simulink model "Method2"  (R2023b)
settings: Solver=FixedStepDiscrete  StartTime=0.0  StopTime=0.5  RelTol=1e-3  EnableMultiTasking=on
undefined symbols (not defined in the file): Datasheet, derived, set
libraries: fl_lib x13, nesl_utility x9, ee_lib x4, slpidlib x1, simulink x1, simulink_extras x1, spspowerguiLib x1

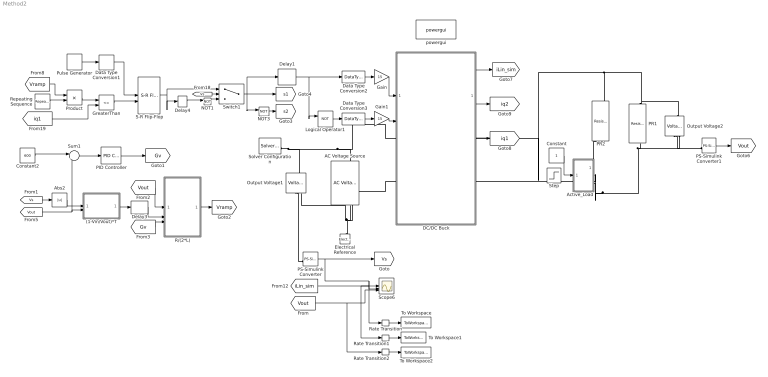
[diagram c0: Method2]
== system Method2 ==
  (1-Vin/Vout)*T : MATLAB Function  TreatAsAtomicUnit=on
  AC Voltage Source : fl_lib/Electrical/Electrical Sources/AC Voltage Source  amp=340 V  shift=0 deg  frequency=50 Hz  omega=0 rad/s
  Abs2 : Abs
  Active_Load : Subsystem
  Constant : Constant
  Constant2 : Constant  Value=600
  DC/DC Buck : Subsystem
  Data Type Conversion1 : DataTypeConversion
  Data Type Conversion2 : DataTypeConversion  OutDataTypeStr=double  RndMeth=Simplest
  Data Type Conversion3 : DataTypeConversion  OutDataTypeStr=double  RndMeth=Simplest
  Delay1 : Delay  DelayLength=1
  Delay3 : Delay  DelayLength=10
  Delay4 : Delay  DelayLength=100e3
  Electrical Reference : fl_lib/Electrical/Electrical Elements/Electrical Reference
  Gain : Gain  Gain=15
  Gain1 : Gain  Gain=15
  GreaterThan : RelationalOperator  Operator=<=  OutDataTypeStr=boolean  RndMeth=Simplest
  Logical Operator1 : Logic  Operator=NOT  AllPortsSameDT=off  OutDataTypeStr=boolean
  NOT1 : Logic  Operator=NOT  IconShape=distinctive  AllPortsSameDT=off  OutDataTypeStr=boolean
  NOT3 : Logic  Operator=NOT  IconShape=distinctive  AllPortsSameDT=off  OutDataTypeStr=boolean
  Output Voltage1 : fl_lib/Electrical/Electrical Sensors/Voltage Sensor  Priority=0
  Output Voltage2 : fl_lib/Electrical/Electrical Sensors/Voltage Sensor  Priority=0
  PID Controller : slpidlib/PID Controller  Controller=PID  Form=Parallel  TimeDomain=Discrete-time  UseExternalTs=off  SampleTime=-1  IntegratorMethod=Forward Euler  FilterMethod=Forward Euler  ControllerParametersSource=internal  P=0  I=0.01  UseKiTs=off  D=0  N=100  UseFilter=on  TunerSelectOption=Transfer Function Based (PID Tuner App)  InitialConditionSource=internal  InitialConditionForIntegrator=0  InitialConditionForFilter=0  DifferentiatorICPrevScaledInput=0  ExternalReset=none  TrackingMode=off  Kt=1  LimitOutput=off  SatLimitsSource=internal  UpperSaturationLimit=0.9  LowerSaturationLimit=0  LinearizeAsGain=on  AntiWindupMode=none  Kb=1  LimitIntegrator=off  UpperIntegratorSaturationLimit=inf  LowerIntegratorSaturationLimit=-inf  POutMin=[]  POutMax=[]  IOutMin=[]  IOutMax=[]  DOutMin=[]  DOutMax=[]  NOutMin=[]  NOutMax=[]  SumOutMin=[]  SumOutMax=[]  SaturationOutMin=[]  SaturationOutMax=[]  PParamMin=[]  PParamMax=[]  IParamMin=[]  IParamMax=[]  DParamMin=[]  DParamMax=[]  NParamMin=[]  NParamMax=[]  KbParamMin=[]  KbParamMax=[]  KtParamMin=[]  KtParamMax=[]  KbOutMin=[]  KbOutMax=[]  KtOutMin=[]  KtOutMax=[]  IntegratorOutMin=[]  IntegratorOutMax=[]  FilterOutMin=[]  FilterOutMax=[]  SumI1OutMin=[]  SumI1OutMax=[]  SumI2OutMin=[]  SumI2OutMax=[]  SumI3OutMin=[]  SumI3OutMax=[]  SumI4OutMin=[]  SumI4OutMax=[]  SumDOutMin=[]  SumDOutMax=[]  DifferentiatorOutMin=[]  DifferentiatorOutMax=[]  FilterDiffOutCoefMin=[]  FilterDiffOutCoefMax=[]  ReciprocalOutMin=[]  ReciprocalOutMax=[]  SumDenOutMin=[]  SumDenOutMax=[]  SumNumOutMin=[]  SumNumOutMax=[]  DivideOutMin=[]  DivideOutMax=[]  UdiffTsProdOutMin=[]  UdiffTsProdOutMax=[]  NTsProdOutMin=[]  NTsProdOutMax=[]  UintegralTsProdOutMin=[]  UintegralTsProdOutMax=[]  UngainTsProdOutMin=[]  UngainTsProdOutMax=[]  ClampingZeroOutDataTypeStr=Inherit: Inherit via back propagation  ClampingZeroOutMin=[]  ClampingZeroOutMax=[]  FilterDenConstantOutDataTypeStr=Inherit: Inherit via back propagation  FilterDenConstantOutMin=[]  FilterDenConstantOutMax=[]  PCopyOutDataTypeStr=Inherit: Inherit via back propagation  PCopyOutMin=[]  PCopyOutMax=[]  NCopyOutDataTypeStr=Inherit: Inherit via back propagation  NCopyOutMin=[]  NCopyOutMax=[]  IntegratorContinuousStateAttributes=''  IntegratorStateMustResolveToSignalObject=off  IntegratorRTWStateStorageClass=Auto  FilterContinuousStateAttributes=''  FilterStateMustResolveToSignalObject=off  FilterRTWStateStorageClass=Auto  ParallelPVariant=InternalParameters  IdealPVariant=Disabled  IVariant=InternalParameters  DVariant=InternalParameters  IntegratorVariant=Discrete  SatVariant=Disabled  AWVariant=Passthrough  PCopyVariant=Disabled  TRVariant=Disabled  FdbkBlocksVariant=Forward  IdealPFdbkVariant=Disabled  SatFdbkVariant=Disabled  DerivativeFilterVariant=ForwardEulerFilter  NVariant=InternalParameters  NCopyVariant=Disabled  FilterICVariant=InternalICsFilter  IntegratorICVariant=InternalICs  ExternalResetVariant=Disabled  TRSumVariant=Passthrough  SumFdbkVariant=Disabled  SumVariant=Sum_PID  TsampFilterVariant=InternalTs  TsampNgainVariant=Passthrough  TsampIntegralVariant=Disabled_SignalSpec  ExternalSaturationOutDataTypeStr=Inherit: Same as second input
  PR1 : fl_lib/Electrical/Electrical Elements/Resistor  R=360 Ohm  i_specify=off  i_priority=None  i=0 A  i_nominal_specify=off  i_nominal_unit=A  i_nominal_value=1  v_specify=off  v_priority=None  v=0 V  v_nominal_specify=off  v_nominal_unit=V  v_nominal_value=1
  PR2 : fl_lib/Electrical/Electrical Elements/Resistor  R=360 Ohm  i_specify=off  i_priority=None  i=0 A  i_nominal_specify=off  i_nominal_unit=A  i_nominal_value=1  v_specify=off  v_priority=None  v=0 V  v_nominal_specify=off  v_nominal_unit=V  v_nominal_value=1
  PS-Simulink Converter : nesl_utility/PS-Simulink Converter  Priority=2  PhysicalDomain=network_engine_domain  SubClassName=ps_output  LeftPortType=input  RightPortType=output  PseudoPeriodic=off  Frequencies=[]  VectorFormat=1-D array  Unit=1  AffineConversion=off
  PS-Simulink Converter1 : nesl_utility/PS-Simulink Converter  Priority=2  PhysicalDomain=network_engine_domain  SubClassName=ps_output  LeftPortType=input  RightPortType=output  PseudoPeriodic=off  Frequencies=[]  VectorFormat=1-D array  Unit=1  AffineConversion=off
  Product : Product
  Pulse Generator : DiscretePulseGenerator  PulseType=Time based  Period=10e-6
  R/(2*L) : MATLAB Function  TreatAsAtomicUnit=on
  Rate Transition : RateTransition  OutPortSampleTime=1e-5
  Rate Transition1 : RateTransition  OutPortSampleTime=1e-5
  Rate Transition2 : RateTransition  OutPortSampleTime=1e-5
  Repeating Sequence : simulink/Sources/Repeating Sequence  rep_seq_t=[0 10e-6]  rep_seq_y=[1 0]
  S-R Flip-Flop : simulink_extras/Flip Flops/S-R Flip-Flop  initial_condition=0
  Scope6 : Scope  NumInputPorts=3
  Solver Configuration : nesl_utility/Solver Configuration  PhysicalDomain=network_engine_domain  SubClassName=solver  LeftPortType=input  RightPortType=generic  Tones=[]  Harmonics=[]  SimulateNoise=off  Profile=off  UseLocalSampling=off  EnableSwitchedLinearOptims=on  FrequencyDomain=off  UseCCode=off  RelTol=0.001  AbsTol=1e-06  MinStep=1e-09  ToWorkspace=off  RevertToSquareIcSolve=off  NumHomotopyIterations=100  PhasorMode=off  PhasorModeNumHarmonics=1  ConsistencySolver=NEWTON_FTOL  IndexReductionMethod=DerivativeReplacement  DoDC=off  ResidualTolerance=1e-08  ConsistencyTolSource=GLOBAL  ConsistencyAbsTol=0.001  ConsistencyRelTol=0.001  ConsistencyTolFactor=0.001  UseLocalSolver=on  LocalSolverChoice=NE_TRAPEZOIDAL_ADVANCER  ResolveIndetEquations=on  FunctionEvalNumThread=1  LocalSolverSampleTime=1e-7  DoFixedCost=on  MaxNonlinIter=3  MaxModeIter=2  ComputeImpulses=off  ImpulseIterations=2  LinearAlgebra=auto  LinearAlgebraNumThread=0  EquationFormulation=NE_TIME_EF  DelaysMemoryBudget=1024  AutomaticFiltering=on  FilteringTimeConstant=0.001  PartitionStorageMethod=AS_NEEDED  PartitionMemoryBudget=1024  PartitionMethod=ROBUST  MultibodyUseLocalSolver=off  MultibodyLocalSolverChoice=ODE1  MultibodyLocalSolverSampleTime=0.001
  Step : Step  Time=0.2  Before=1  After=0  SampleTime=0
  Sum1 : Sum  Inputs=|+-
  Switch1 : Switch  Criteria=u2 > Threshold
  To Workspace : ToWorkspace  VariableName=Vs_method2  SaveFormat=Timeseries  SampleTime=-1
  To Workspace1 : ToWorkspace  VariableName=I_method2  SaveFormat=Timeseries  SampleTime=-1
  To Workspace2 : ToWorkspace  VariableName=Vout_method2  SaveFormat=Timeseries  SampleTime=-1
  powergui : spspowerguiLib/powergui  Priority=1  SimulationMode=Continuous  SampleTime=1e-6  frequency=60  Iterations=50  frequencyindice=60  Pbase=100e6  ErrMax=1e-4  UnitsV=kV  UnitsW=MW  buscounter=0  FunctionMessages=off  echomessages=off  EnableUseOfTLC=off  CurrentSourceSwitches=off  DisableSnubberDevices=off  DisableRonSwitches=off  DisableVfSwitches=off  DisplayEquations=off  AutomaticDiscreteSolvers=off  SolverType=Tustin/Backward Euler (TBE)  Interpol=off  ExternalGateDelay=off  methode=off  Ts=100  x0status=blocks  SPID=on  SwTol=0  HookPort=off  NonlinearTolerance=1e-4  nMaxIteration=100  ContinueOnMaxIteration=off  RestoreLinks=warning  ResistiveCurrentMeasurement=off  Frange=[0:2:500]  Ylog=off  Xlog=on  ShowGrid=off  save=off  variable=ZData  structure=0  ZoomFFT=off  StartTime=0.0  cycles=1  DisplayStyle=1  fundamental=60  FreqAxis=off  MaxFrequency=1000  frequencyindicesteady=1  RmsSteady=1  display=off
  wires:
  Logical Operator1/1 -> Data Type Conversion3/1
  DC/DC Buck/1(I_sensor) -> [iLin_sim]
  Switch1/1 -> Delay1/1, NOT3/1, [s1]
  [iLin_sim] -> Rate Transition1/1, Scope6/2
  S-R Flip-Flop/1 -> Switch1/1, Delay4/1
  NOT3/1 -> [s2]
  GreaterThan/1 -> S-R Flip-Flop/2
  Delay4/1 -> NOT1/1
  [Vs] -> Switch1/2
  Data Type Conversion1/1 -> S-R Flip-Flop/1
  Pulse Generator/1 -> Data Type Conversion1/1
  Repeating Sequence/1 -> Product/2
  Product/1 -> GreaterThan/1
  PS-Simulink Converter/1 -> [Vs], Rate Transition/1, Scope6/1
  (1-Vin/Vout)*T/1(Ton) -> Delay3/1
  [Gv] -> R/(2*L)/3(Gv)
  Delay3/1 -> R/(2*L)/2(Ton)
  R/(2*L)/1(y) -> [Vramp]
  PID Controller/1 -> [Gv]
  Sum1/1 -> PID Controller/1
  [Vs] -> Abs2/1
  [Vout] -> R/(2*L)/1(Vout)
  Constant2/1 -> Sum1/1
  [Vramp] -> Product/1
  [Vout] -> (1-Vin/Vout)*T/2(Vout), Sum1/2
  PS-Simulink Converter1/1 -> [Vout]
  Abs2/1 -> (1-Vin/Vout)*T/1(Vin)
  [iq1] -> GreaterThan/2
  DC/DC Buck/3(iq1) -> [iq1]
  DC/DC Buck/2(iq2) -> [iq2]
  NOT1/1 -> Switch1/3
  Delay1/1 -> Data Type Conversion2/1, Logical Operator1/1
  [Vout] -> Rate Transition2/1, Scope6/3
  Rate Transition/1 -> To Workspace/1
  Rate Transition1/1 -> To Workspace1/1
  Rate Transition2/1 -> To Workspace2/1
  Gain/1 -> DC/DC Buck/1(In1)
  Data Type Conversion2/1 -> Gain/1
  Gain1/1 -> DC/DC Buck/2(In2)
  Data Type Conversion3/1 -> Gain1/1
  Constant/1 -> Active_Load/1(In1)
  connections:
  Output Voltage2/RConn2 -- PR1/RConn1 -- Active_Load/RConn2 -- DC/DC Buck/RConn2
  Solver Configuration/RConn1 -- AC Voltage Source/LConn1 -- DC/DC Buck/LConn1 -- Output Voltage1/LConn1
  Electrical Reference/LConn1 -- DC/DC Buck/LConn2 -- Output Voltage1/RConn2 -- AC Voltage Source/RConn1
  Output Voltage2/LConn1 -- PR1/LConn1 -- PR2/LConn1 -- DC/DC Buck/RConn1
  Active_Load/RConn1 -- PR2/RConn1
  PS-Simulink Converter/LConn1 -- Output Voltage1/RConn1
  PS-Simulink Converter1/LConn1 -- Output Voltage2/RConn1

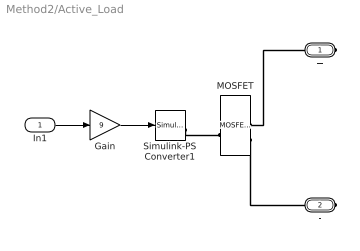
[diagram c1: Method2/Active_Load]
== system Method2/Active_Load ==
  In1 : Inport
  Gain : Gain  Gain=9
  MOSFET : ee_lib/Semiconductors & Converters/MOSFET (Ideal, Switching)  port_option=ee.enum.controlport.ps  Rds=0.2 Ohm  Goff=1e-6 1/Ohm  Vth=3 V  diode_param=2  diode_Vf=1.6 V  diode_Ron=0.001 Ohm  diode_Goff=1e-5 1/Ohm  diode_C=5e-8 F  diode_iRM=-235 A  diode_iF=300 A  diode_idot=-100 A/us  diode_trr_param=2  diode_trr_factor=3  diode_trr=70 ns  diode_Qrr=1.5e+3 s*uA  ids_specify=off  ids_priority=None  ids=0 A  ids_nominal_specify=off  ids_nominal_unit=A  ids_nominal_value=1  vds_specify=off  vds_priority=None  vds=0 V  vds_nominal_specify=off  vds_nominal_unit=V  vds_nominal_value=1  vgs_specify=off  vgs_priority=None  vgs=0 V  vgs_nominal_specify=off  vgs_nominal_unit=V  vgs_nominal_value=1  thermal_loss_option=ee.enum.converters.thermalLossOption.constantvalues  Von_data=[0, 1.8, 3.2, 6, 10, 16; 0, 2, 5.5, 9.5, 15, 25] V  Tj=[298.15, 448.15] K  Iout_data=[0, 20, 40, 60, 80, 100] A  Eon_data=[0, 55.04, 124.57, 235.53, 362.12; 0, 71.25, 161.25, 304.88, 468.75] * 1e-6 J  Eoff_data=[0, 18, 30, 56.1, 76.5; 0, 22.5, 37.5, 70.13, 95.63] * 1e-6 J  Eon_data_3D=[zeros(2, 5, 3)] J  Eoff_data_3D=[zeros(2, 5, 3)] J  Tj_loss=[298.15, 448.15] K  Iout_data_loss=[0, 10, 20, 30, 40] A  tabulateWithVds=false  Vds_loss=[0, 150, 300] V  Eon_scalar=22.86e-3 J  Eoff_scalar=17.14e-3 J  Voff=300 V  Iout_scalar=600 A  useCurrentFromPreviousCycle=false  useVoltageFromPreviousCycle=false  diodeModelType=ee.enum.converters.diodeModelType.pwl  diodeTableType=ee.enum.diode.tableType.IfMat  diode_IfMat=[.07, .12, .19, 1.75, 4.24, 7.32, 11.2; .16, .3, .72, 2.14, 4.02, 6.35, 9.12] A  diode_VfMat=[.9, 1.15, 1.25, 1.5, 1.75, 2.17, 2.6, 2.85; .58, .68, .75, 1.1, 1.38, 1.77, 2.27, 2.7] V  diode_TjVec=[25, 125] degC  diode_VfVec=[.5, .7, .9, 1.3, 1.7, 2.1, 2.5] V  diode_IfVec=[.1, .2, .5, 1, 2, 4, 7, 10] A  diode_Vr=-600 V  diode_Ls=150 nH  diode_Erec=0.03 J  diode_rec_loss_model=ee.enum.diode.reverseRecoveryModel.fixed  diode_ErecVal=0 J  diode_scaleWithIandV=true  diode_ErecMat=zeros(2, 3) J  diode_TjrecVec=[298.15, 398.15] K  diode_IfrecVec=[.1, 1, 10] A  diode_IrecVal=10 A  diode_VrecVal=10 V  diode_tFilter=1 / 1000 / 100 s  thermal_network_parameterization=ee.enum.thermalNetworkTopology.external  Rth=[.03, .2] K/W  Rth_Cauer=[.03, .1, .2] K/W  Rth_Foster=[.03, .2] K/W  thermal_mass_parameterization=ee.enum.thermalNetwork.timeconstant  thermal_mass=[3, 25] J/K  thermal_mass_Cauer=[3, 10, 25] J/K  thermal_mass_Foster=[33, 50] J/K  thermal_time_constant=[.1, 5] s  thermal_time_constant_Cauer=[.1, 1, 5] s  thermal_time_constant_Foster=[1, 10] s  thermal_mass_initial_temperatures=[25, 25] degC  thermal_mass_initial_temperatures_Cauer=[25, 25, 25] degC  junction_thermal_mass=0.1 J/K  Tvec_initial_Foster=[25, 25, 25, 25] degC  no_thermal_network=0  junction_temperature_specify=off  junction_temperature_priority=None  junction_temperature=25 degC  junction_temperature_nominal_specify=off  junction_temperature_nominal_unit=degC  junction_temperature_nominal_value=1  Qj_specify=off  Qj_priority=None  Qj=0 W  Qj_nominal_specify=off  Qj_nominal_unit=W  Qj_nominal_value=1  accumulatedSwitchingLosses_specify=off  accumulatedSwitchingLosses_priority=None  accumulatedSwitchingLosses=0 J
  Simulink-PS Converter1 : nesl_utility/Simulink-PS Converter  PhysicalDomain=network_engine_domain  SubClassName=ps_input  LeftPortType=input  RightPortType=output  PseudoPeriodic=off  Frequencies=[]  NoiseDistribution=none  NoiseParameters=[]  Unit=1  AffineConversion=off  FilteringAndDerivatives=provide  SimscapeFilterOrder=1  InputFilterTimeConstant=0.001  UdotUserProvided=0
  + : PMIOPort  Side=Right
  - : PMIOPort  Port=2  Side=Right
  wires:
  In1/1 -> Gain/1
  Gain/1 -> Simulink-PS Converter1/1
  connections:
  MOSFET/RConn2 -- -/RConn1
  MOSFET/RConn1 -- +/RConn1
  Simulink-PS Converter1/RConn1 -- MOSFET/LConn1

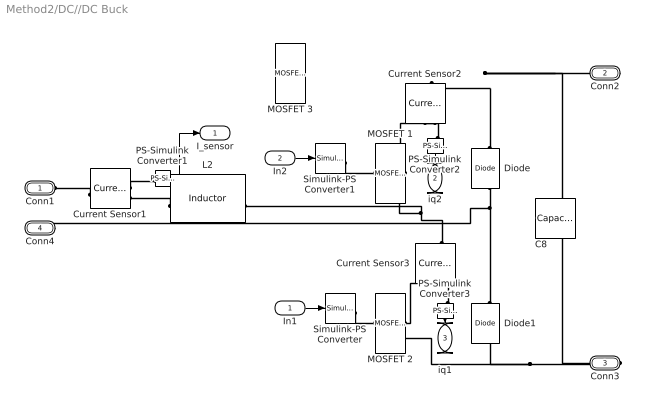
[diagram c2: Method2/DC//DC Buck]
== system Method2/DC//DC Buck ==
  In1 : Inport
  In2 : Inport  Port=2
  C8 : fl_lib/Electrical/Electrical Elements/Capacitor  c=0.1 mF  r=0.15 Ohm  g=0 1/Ohm  i_specify=off  i_priority=None  i=0 A  i_nominal_specify=off  i_nominal_unit=A  i_nominal_value=1  v_specify=off  v_priority=None  v=0 V  v_nominal_specify=off  v_nominal_unit=V  v_nominal_value=1  vc_specify=on  vc_priority=High  vc=0 V  vc_nominal_specify=off  vc_nominal_unit=V  vc_nominal_value=1
  Current Sensor1 : fl_lib/Electrical/Electrical Sensors/Current Sensor
  Current Sensor2 : fl_lib/Electrical/Electrical Sensors/Current Sensor
  Current Sensor3 : fl_lib/Electrical/Electrical Sensors/Current Sensor
  Diode : fl_lib/Electrical/Electrical Elements/Diode  Vf=0.6 V  Ron=0.3 Ohm  Goff=1e-8 1/Ohm  i_specify=off  i_priority=None  i=0 A  i_nominal_specify=off  i_nominal_unit=A  i_nominal_value=1  v_specify=off  v_priority=None  v=0 V  v_nominal_specify=off  v_nominal_unit=V  v_nominal_value=1
  Diode1 : fl_lib/Electrical/Electrical Elements/Diode  Vf=0.6 V  Ron=0.3 Ohm  Goff=1e-8 1/Ohm  i_specify=off  i_priority=None  i=0 A  i_nominal_specify=off  i_nominal_unit=A  i_nominal_value=1  v_specify=off  v_priority=None  v=0 V  v_nominal_specify=off  v_nominal_unit=V  v_nominal_value=1
  L2 : fl_lib/Electrical/Electrical Elements/Inductor  l=1 mH  r=0.0105 Ohm  g=0 1/Ohm  i_specify=off  i_priority=None  i=0 A  i_nominal_specify=off  i_nominal_unit=A  i_nominal_value=1  v_specify=off  v_priority=None  v=0 V  v_nominal_specify=off  v_nominal_unit=V  v_nominal_value=1  i_L_specify=off  i_L_priority=High  i_L=0 A  i_L_nominal_specify=off  i_L_nominal_unit=A  i_L_nominal_value=1
  MOSFET 1 : ee_lib/Semiconductors & Converters/MOSFET (Ideal, Switching)  Tag={'toolbox/physmod/elec/library/m/ee_lib_parts';'Semiconductors_and_Converters/MOSFET__Ideal__Switching_/Infineon/AIMW120R080M1.xml'}  port_option=ee.enum.controlport.ps  Rds=0.26 % Datasheet derived Ohm  Goff=2e-08 % Datasheet derived 1/Ohm  Vth=4.5 % Datasheet derived V  diode_param=ee.enum.converters.protectiondiode.nodynamics  diode_Vf=3.83 % Datasheet derived V  diode_Ron=0.048 % Datasheet derived Ohm  diode_Goff=1e-05 % Library default 1/Ohm  diode_C=50e-9 % Parameter not set F  diode_iRM=-235 % Parameter not set A  diode_iF=300 % Parameter not set A  diode_idot=-50 % Parameter not set A/us  diode_trr_param=ee.enum.converters.diodeReverseParam.trr_factor  diode_trr_factor=3 % Parameter not set  diode_trr=15 % Parameter not set us  diode_Qrr=1500 % Parameter not set s*uA  ids_specify=off  ids_priority=None  ids=0 A  ids_nominal_specify=off  ids_nominal_unit=A  ids_nominal_value=1  vds_specify=off  vds_priority=None  vds=0 V  vds_nominal_specify=off  vds_nominal_unit=V  vds_nominal_value=1  vgs_specify=off  vgs_priority=None  vgs=0 V  vgs_nominal_specify=off  vgs_nominal_unit=V  vgs_nominal_value=1  thermal_loss_option=ee.enum.converters.thermalLossOption.tabulated2d  Von_data=[0 0.21 0.42 0.63 0.84 1.22 1.66 2.09 2.57 3.09 3.61 4.18 4.91 5.65 6.38 7.33 8.31 9.43 10.71 12 13.81 15.69 17.78 19.87;0 0.41 0.81 1.22 1.63 2.03 2.59 3.16 3.72 4.29 4.99 5.68 6.4 7.26 8.12 8.98 10.07 11.23 12.38 13.89 15.4 17 18.83 20.65] % Datasheet derived V  Tj=[25 175] % Datasheet derived degC  Iout_data=[0 3.3 6.6 9.9 13.2 16.5 19.8 23.1 26.4 29.71 33.01 36.31 39.61 42.91 46.21 49.51 52.81 56.11 59.41 62.71 66.01 69.31 72.61 75.91] % Datasheet derived A  Eon_data=[0 2.39 17.04 31.69 46.33 60.98 75.63 90.28 104.92 119.57 134.22 148.87 163.51 178.16 192.81 207.46 222.1 236.75 251.37 265.31 279.25 293.19 307.13 321.07 335.01 348.95 362.89 376.83 390.77 405.86 424.27 442.67 461.07 479.48 497.88 517.66 543.15 568.63 594.12 619.6 645.09 670.57 696.06 721.54 747.83 777.14 806.45 835.76 865.07 894.38 923.69 953 982.31 1011.52 1040.61 1069.7 1098.79 1127.88 1156.96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  Eoff_data=[84.71 85.86 87.02 88.18 89.33 90.49 91.65 92.8 93.96 95.12 96.28 97.43 98.59 99.75 100.9 102.06 103.22 104.37 105.53 106.69 107.84 109 110.16 111.32 112.47 113.63 114.79 116.16 118 119.85 121.69 123.53 125.38 127.22 129.07 130.91 132.75 134.6 136.44 138.28 140.13 141.97 145.4 149.39 153.38 157.37 161.36 165.36 169.35 173.34 177.33 181.32 185.32 189.31 193.3 197.29 201.29 205.28 209.27 213.26 217.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  Eon_data_3D=[zeros(2, 5, 3)] % Parameter not set J  Eoff_data_3D=[zeros(2, 5, 3)] % Parameter not set J  Tj_loss=175 % Datasheet derived degC  Iout_data_loss=[0 0.55 1.11 1.66 2.22 2.77 3.33 3.88 4.43 4.99 5.54 6.1 6.65 7.2 7.76 8.31 8.87 9.42 9.98 10.53 11.08 11.64 12.19 12.75 13.3 13.86 14.41 14.96 15.52 16.07 16.63 17.18 17.74 18.29 18.84 19.4 19.95 20.51 21.06 21.61 22.17 22.72 23.28 23.83 24.39 24.94 25.49 26.05 26.6 27.16 27.71 28.27 28.82 29.37 29.93 30.48 31.04 31.59 32.15 32.7 33.25 33.81 34.36 34.92 35.47 36.02 36.58 37.13 37.69 38.24 38.8 39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  tabulateWithVds=false % Parameter not set  Vds_loss=[0, 150, 300] % Parameter not set V  Eon_scalar=22.86e-3 % Parameter not set J  Eoff_scalar=17.14e-3 % Parameter not set J  Voff=800 % Datasheet derived V  Iout_scalar=600 % Parameter not set A  useCurrentFromPreviousCycle=false  useVoltageFromPreviousCycle=false  diodeModelType=ee.enum.converters.diodeModelType.tabulated  diodeTableType=ee.enum.diode.tableType.IfMat  diode_IfMat=[0 0.102 0.2053 0.3102 3.8793 10.0341 16.4314 29.8;0 0.0638 0.4957 1.6585 6.589 12.4788 21.029 38.7605] % Datasheet derived A  diode_VfMat=[.9, 1.15, 1.25, 1.5, 1.75, 2.17, 2.6, 2.85; .58, .68, .75, 1.1, 1.38, 1.77, 2.27, 2.7] % Parameter not set V  diode_TjVec=[25 175] % Datasheet derived degC  diode_VfVec=[0 0.7 1.4 2.1 2.81 3.51 4.21 4.91] % Datasheet derived V  diode_IfVec=[.1, .2, .5, 1, 2, 4, 7, 10] % Parameter not set A  diode_Vr=-600 % Parameter not set V  diode_Ls=150 % Parameter not set nH  diode_Erec=0.03 % Parameter not set J  diode_rec_loss_model=ee.enum.diode.reverseRecoveryModel.fixed  diode_ErecVal=0 % Parameter not set J  diode_scaleWithIandV=false  diode_ErecMat=zeros(2, 3) % Parameter not set J  diode_TjrecVec=[298.15, 398.15] % Parameter not set K  diode_IfrecVec=[.1, 1, 10] % Parameter not set A  diode_IrecVal=10 % Parameter not set A  diode_VrecVal=10 % Parameter not set V  diode_tFilter=1 / 1000 / 100 % Parameter not set s  thermal_network_parameterization=ee.enum.thermalNetworkTopology.cauer  Rth=[.03, .2] % Parameter not set K/W  Rth_Cauer=[.03, .1, .2] % Parameter not set K/W  Rth_Foster=[.03, .2] % Parameter not set K/W  thermal_mass_parameterization=ee.enum.thermalNetwork.timeconstant  thermal_mass=[3, 25] % Parameter not set J/K  thermal_mass_Cauer=[3, 10, 25] % Parameter not set J/K  thermal_mass_Foster=[33, 50] % Parameter not set J/K  thermal_time_constant=[.1, 5] % Parameter not set s  thermal_time_constant_Cauer=[.1, 1, 5] % Parameter not set s  thermal_time_constant_Foster=[1, 10] % Parameter not set s  thermal_mass_initial_temperatures=[25, 25] % Parameter not set degC  thermal_mass_initial_temperatures_Cauer=[25, 25, 25] % Parameter not set degC  junction_thermal_mass=4.04 % Datasheet derived J/K  Tvec_initial_Foster=[25, 25, 25, 25] % Parameter not set degC  no_thermal_network=0 % Parameter not set  junction_temperature_specify=off  junction_temperature_priority=None  junction_temperature=25 degC  junction_temperature_nominal_specify=off  junction_temperature_nominal_unit=degC  junction_temperature_nominal_value=1  Qj_specify=off  Qj_priority=None  Qj=0 W  Qj_nominal_specify=off  Qj_nominal_unit=W  Qj_nominal_value=1  accumulatedSwitchingLosses_specify=off  accumulatedSwitchingLosses_priority=None  accumulatedSwitchingLosses=0 J
  MOSFET 2 : ee_lib/Semiconductors & Converters/MOSFET (Ideal, Switching)  Tag={'toolbox/physmod/elec/library/m/ee_lib_parts';'Semiconductors_and_Converters/MOSFET__Ideal__Switching_/Infineon/AIMW120R080M1.xml'}  port_option=ee.enum.controlport.ps  Rds=0.26 % Datasheet derived Ohm  Goff=2e-08 % Datasheet derived 1/Ohm  Vth=4.5 % Datasheet derived V  diode_param=ee.enum.converters.protectiondiode.nodynamics  diode_Vf=3.83 % Datasheet derived V  diode_Ron=0.048 % Datasheet derived Ohm  diode_Goff=1e-05 % Library default 1/Ohm  diode_C=50e-9 % Parameter not set F  diode_iRM=-235 % Parameter not set A  diode_iF=300 % Parameter not set A  diode_idot=-50 % Parameter not set A/us  diode_trr_param=ee.enum.converters.diodeReverseParam.trr_factor  diode_trr_factor=3 % Parameter not set  diode_trr=15 % Parameter not set us  diode_Qrr=1500 % Parameter not set s*uA  ids_specify=off  ids_priority=None  ids=0 A  ids_nominal_specify=off  ids_nominal_unit=A  ids_nominal_value=1  vds_specify=off  vds_priority=None  vds=0 V  vds_nominal_specify=off  vds_nominal_unit=V  vds_nominal_value=1  vgs_specify=off  vgs_priority=None  vgs=0 V  vgs_nominal_specify=off  vgs_nominal_unit=V  vgs_nominal_value=1  thermal_loss_option=ee.enum.converters.thermalLossOption.tabulated2d  Von_data=[0 0.21 0.42 0.63 0.84 1.22 1.66 2.09 2.57 3.09 3.61 4.18 4.91 5.65 6.38 7.33 8.31 9.43 10.71 12 13.81 15.69 17.78 19.87;0 0.41 0.81 1.22 1.63 2.03 2.59 3.16 3.72 4.29 4.99 5.68 6.4 7.26 8.12 8.98 10.07 11.23 12.38 13.89 15.4 17 18.83 20.65] % Datasheet derived V  Tj=[25 175] % Datasheet derived degC  Iout_data=[0 3.3 6.6 9.9 13.2 16.5 19.8 23.1 26.4 29.71 33.01 36.31 39.61 42.91 46.21 49.51 52.81 56.11 59.41 62.71 66.01 69.31 72.61 75.91] % Datasheet derived A  Eon_data=[0 2.39 17.04 31.69 46.33 60.98 75.63 90.28 104.92 119.57 134.22 148.87 163.51 178.16 192.81 207.46 222.1 236.75 251.37 265.31 279.25 293.19 307.13 321.07 335.01 348.95 362.89 376.83 390.77 405.86 424.27 442.67 461.07 479.48 497.88 517.66 543.15 568.63 594.12 619.6 645.09 670.57 696.06 721.54 747.83 777.14 806.45 835.76 865.07 894.38 923.69 953 982.31 1011.52 1040.61 1069.7 1098.79 1127.88 1156.96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  Eoff_data=[84.71 85.86 87.02 88.18 89.33 90.49 91.65 92.8 93.96 95.12 96.28 97.43 98.59 99.75 100.9 102.06 103.22 104.37 105.53 106.69 107.84 109 110.16 111.32 112.47 113.63 114.79 116.16 118 119.85 121.69 123.53 125.38 127.22 129.07 130.91 132.75 134.6 136.44 138.28 140.13 141.97 145.4 149.39 153.38 157.37 161.36 165.36 169.35 173.34 177.33 181.32 185.32 189.31 193.3 197.29 201.29 205.28 209.27 213.26 217.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  Eon_data_3D=[zeros(2, 5, 3)] % Parameter not set J  Eoff_data_3D=[zeros(2, 5, 3)] % Parameter not set J  Tj_loss=175 % Datasheet derived degC  Iout_data_loss=[0 0.55 1.11 1.66 2.22 2.77 3.33 3.88 4.43 4.99 5.54 6.1 6.65 7.2 7.76 8.31 8.87 9.42 9.98 10.53 11.08 11.64 12.19 12.75 13.3 13.86 14.41 14.96 15.52 16.07 16.63 17.18 17.74 18.29 18.84 19.4 19.95 20.51 21.06 21.61 22.17 22.72 23.28 23.83 24.39 24.94 25.49 26.05 26.6 27.16 27.71 28.27 28.82 29.37 29.93 30.48 31.04 31.59 32.15 32.7 33.25 33.81 34.36 34.92 35.47 36.02 36.58 37.13 37.69 38.24 38.8 39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  tabulateWithVds=false % Parameter not set  Vds_loss=[0, 150, 300] % Parameter not set V  Eon_scalar=22.86e-3 % Parameter not set J  Eoff_scalar=17.14e-3 % Parameter not set J  Voff=800 % Datasheet derived V  Iout_scalar=600 % Parameter not set A  useCurrentFromPreviousCycle=false  useVoltageFromPreviousCycle=false  diodeModelType=ee.enum.converters.diodeModelType.tabulated  diodeTableType=ee.enum.diode.tableType.IfMat  diode_IfMat=[0 0.102 0.2053 0.3102 3.8793 10.0341 16.4314 29.8;0 0.0638 0.4957 1.6585 6.589 12.4788 21.029 38.7605] % Datasheet derived A  diode_VfMat=[.9, 1.15, 1.25, 1.5, 1.75, 2.17, 2.6, 2.85; .58, .68, .75, 1.1, 1.38, 1.77, 2.27, 2.7] % Parameter not set V  diode_TjVec=[25 175] % Datasheet derived degC  diode_VfVec=[0 0.7 1.4 2.1 2.81 3.51 4.21 4.91] % Datasheet derived V  diode_IfVec=[.1, .2, .5, 1, 2, 4, 7, 10] % Parameter not set A  diode_Vr=-600 % Parameter not set V  diode_Ls=150 % Parameter not set nH  diode_Erec=0.03 % Parameter not set J  diode_rec_loss_model=ee.enum.diode.reverseRecoveryModel.fixed  diode_ErecVal=0 % Parameter not set J  diode_scaleWithIandV=false  diode_ErecMat=zeros(2, 3) % Parameter not set J  diode_TjrecVec=[298.15, 398.15] % Parameter not set K  diode_IfrecVec=[.1, 1, 10] % Parameter not set A  diode_IrecVal=10 % Parameter not set A  diode_VrecVal=10 % Parameter not set V  diode_tFilter=1 / 1000 / 100 % Parameter not set s  thermal_network_parameterization=ee.enum.thermalNetworkTopology.cauer  Rth=[.03, .2] % Parameter not set K/W  Rth_Cauer=[.03, .1, .2] % Parameter not set K/W  Rth_Foster=[.03, .2] % Parameter not set K/W  thermal_mass_parameterization=ee.enum.thermalNetwork.timeconstant  thermal_mass=[3, 25] % Parameter not set J/K  thermal_mass_Cauer=[3, 10, 25] % Parameter not set J/K  thermal_mass_Foster=[33, 50] % Parameter not set J/K  thermal_time_constant=[.1, 5] % Parameter not set s  thermal_time_constant_Cauer=[.1, 1, 5] % Parameter not set s  thermal_time_constant_Foster=[1, 10] % Parameter not set s  thermal_mass_initial_temperatures=[25, 25] % Parameter not set degC  thermal_mass_initial_temperatures_Cauer=[25, 25, 25] % Parameter not set degC  junction_thermal_mass=4.04 % Datasheet derived J/K  Tvec_initial_Foster=[25, 25, 25, 25] % Parameter not set degC  no_thermal_network=0 % Parameter not set  junction_temperature_specify=off  junction_temperature_priority=None  junction_temperature=25 degC  junction_temperature_nominal_specify=off  junction_temperature_nominal_unit=degC  junction_temperature_nominal_value=1  Qj_specify=off  Qj_priority=None  Qj=0 W  Qj_nominal_specify=off  Qj_nominal_unit=W  Qj_nominal_value=1  accumulatedSwitchingLosses_specify=off  accumulatedSwitchingLosses_priority=None  accumulatedSwitchingLosses=0 J
  MOSFET 3 : ee_lib/Semiconductors & Converters/MOSFET (Ideal, Switching)  Tag={'toolbox/physmod/elec/library/m/ee_lib_parts';'Semiconductors_and_Converters/MOSFET__Ideal__Switching_/Infineon/AIMW120R080M1.xml'}  port_option=ee.enum.controlport.ps  Rds=0.26 % Datasheet derived Ohm  Goff=2e-08 % Datasheet derived 1/Ohm  Vth=4.5 % Datasheet derived V  diode_param=ee.enum.converters.protectiondiode.nodynamics  diode_Vf=3.83 % Datasheet derived V  diode_Ron=0.048 % Datasheet derived Ohm  diode_Goff=1e-05 % Library default 1/Ohm  diode_C=50e-9 % Parameter not set F  diode_iRM=-235 % Parameter not set A  diode_iF=300 % Parameter not set A  diode_idot=-50 % Parameter not set A/us  diode_trr_param=ee.enum.converters.diodeReverseParam.trr_factor  diode_trr_factor=3 % Parameter not set  diode_trr=15 % Parameter not set us  diode_Qrr=1500 % Parameter not set s*uA  ids_specify=off  ids_priority=None  ids=0 A  ids_nominal_specify=off  ids_nominal_unit=A  ids_nominal_value=1  vds_specify=off  vds_priority=None  vds=0 V  vds_nominal_specify=off  vds_nominal_unit=V  vds_nominal_value=1  vgs_specify=off  vgs_priority=None  vgs=0 V  vgs_nominal_specify=off  vgs_nominal_unit=V  vgs_nominal_value=1  thermal_loss_option=ee.enum.converters.thermalLossOption.constantvalues  Von_data=[0, 1.8, 3.2, 6, 10, 16; 0, 2, 5.5, 9.5, 15, 25] V  Tj=[298.15, 448.15] K  Iout_data=[0, 20, 40, 60, 80, 100] A  Eon_data=[0, 55.04, 124.57, 235.53, 362.12; 0, 71.25, 161.25, 304.88, 468.75] * 1e-6 J  Eoff_data=[0, 18, 30, 56.1, 76.5; 0, 22.5, 37.5, 70.13, 95.63] * 1e-6 J  Eon_data_3D=[zeros(2, 5, 3)] J  Eoff_data_3D=[zeros(2, 5, 3)] J  Tj_loss=[298.15, 448.15] K  Iout_data_loss=[0, 10, 20, 30, 40] A  tabulateWithVds=false  Vds_loss=[0, 150, 300] V  Eon_scalar=22.86e-3 J  Eoff_scalar=17.14e-3 J  Voff=300 V  Iout_scalar=600 A  useCurrentFromPreviousCycle=false  useVoltageFromPreviousCycle=false  diodeModelType=ee.enum.converters.diodeModelType.pwl  diodeTableType=ee.enum.diode.tableType.IfMat  diode_IfMat=[.07, .12, .19, 1.75, 4.24, 7.32, 11.2; .16, .3, .72, 2.14, 4.02, 6.35, 9.12] A  diode_VfMat=[.9, 1.15, 1.25, 1.5, 1.75, 2.17, 2.6, 2.85; .58, .68, .75, 1.1, 1.38, 1.77, 2.27, 2.7] V  diode_TjVec=[25, 125] degC  diode_VfVec=[.5, .7, .9, 1.3, 1.7, 2.1, 2.5] V  diode_IfVec=[.1, .2, .5, 1, 2, 4, 7, 10] A  diode_Vr=-600 V  diode_Ls=150 nH  diode_Erec=0.03 J  diode_rec_loss_model=ee.enum.diode.reverseRecoveryModel.fixed  diode_ErecVal=0 J  diode_scaleWithIandV=true  diode_ErecMat=zeros(2, 3) J  diode_TjrecVec=[298.15, 398.15] K  diode_IfrecVec=[.1, 1, 10] A  diode_IrecVal=10 A  diode_VrecVal=10 V  diode_tFilter=1 / 1000 / 100 s  thermal_network_parameterization=ee.enum.thermalNetworkTopology.external  Rth=[.03, .2] K/W  Rth_Cauer=[.03, .1, .2] K/W  Rth_Foster=[.03, .2] K/W  thermal_mass_parameterization=ee.enum.thermalNetwork.timeconstant  thermal_mass=[3, 25] J/K  thermal_mass_Cauer=[3, 10, 25] J/K  thermal_mass_Foster=[33, 50] J/K  thermal_time_constant=[.1, 5] s  thermal_time_constant_Cauer=[.1, 1, 5] s  thermal_time_constant_Foster=[1, 10] s  thermal_mass_initial_temperatures=[25, 25] degC  thermal_mass_initial_temperatures_Cauer=[25, 25, 25] degC  junction_thermal_mass=0.1 J/K  Tvec_initial_Foster=[25, 25, 25, 25] degC  no_thermal_network=0  junction_temperature_specify=off  junction_temperature_priority=None  junction_temperature=25 degC  junction_temperature_nominal_specify=off  junction_temperature_nominal_unit=degC  junction_temperature_nominal_value=1  Qj_specify=off  Qj_priority=None  Qj=0 W  Qj_nominal_specify=off  Qj_nominal_unit=W  Qj_nominal_value=1  accumulatedSwitchingLosses_specify=off  accumulatedSwitchingLosses_priority=None  accumulatedSwitchingLosses=0 J
  PS-Simulink Converter1 : nesl_utility/PS-Simulink Converter  PhysicalDomain=network_engine_domain  SubClassName=ps_output  LeftPortType=input  RightPortType=output  PseudoPeriodic=off  Frequencies=[]  VectorFormat=inherit  Unit=inherit  AffineConversion=off
  PS-Simulink Converter2 : nesl_utility/PS-Simulink Converter  PhysicalDomain=network_engine_domain  SubClassName=ps_output  LeftPortType=input  RightPortType=output  PseudoPeriodic=off  Frequencies=[]  VectorFormat=inherit  Unit=inherit  AffineConversion=off
  PS-Simulink Converter3 : nesl_utility/PS-Simulink Converter  PhysicalDomain=network_engine_domain  SubClassName=ps_output  LeftPortType=input  RightPortType=output  PseudoPeriodic=off  Frequencies=[]  VectorFormat=inherit  Unit=inherit  AffineConversion=off
  Simulink-PS Converter : nesl_utility/Simulink-PS Converter  PhysicalDomain=network_engine_domain  SubClassName=ps_input  LeftPortType=input  RightPortType=output  PseudoPeriodic=off  Frequencies=[]  NoiseDistribution=none  NoiseParameters=[]  Unit=1  AffineConversion=off  FilteringAndDerivatives=provide  SimscapeFilterOrder=1  InputFilterTimeConstant=0.001  UdotUserProvided=0
  Simulink-PS Converter1 : nesl_utility/Simulink-PS Converter  PhysicalDomain=network_engine_domain  SubClassName=ps_input  LeftPortType=input  RightPortType=output  PseudoPeriodic=off  Frequencies=[]  NoiseDistribution=none  NoiseParameters=[]  Unit=1  AffineConversion=off  FilteringAndDerivatives=provide  SimscapeFilterOrder=1  InputFilterTimeConstant=0.001  UdotUserProvided=0
  Conn1 : PMIOPort  Side=Left
  Conn2 : PMIOPort  Port=2  Side=Right
  Conn3 : PMIOPort  Port=3  Side=Right
  Conn4 : PMIOPort  Port=4  Side=Left
  I_sensor : Outport  VectorParamsAs1DForOutWhenUnconnected=off
  iq2 : Outport  Port=2  VectorParamsAs1DForOutWhenUnconnected=off
  iq1 : Outport  Port=3  VectorParamsAs1DForOutWhenUnconnected=off
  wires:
  In2/1 -> Simulink-PS Converter1/1
  In1/1 -> Simulink-PS Converter/1
  PS-Simulink Converter1/1 -> I_sensor/1
  PS-Simulink Converter3/1 -> iq1/1
  PS-Simulink Converter2/1 -> iq2/1
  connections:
  Conn3/RConn1 -- MOSFET 2/RConn2 -- Diode1/LConn1 -- C8/RConn1
  Simulink-PS Converter1/RConn1 -- MOSFET 1/LConn1
  Current Sensor3/LConn1 -- MOSFET 1/RConn2 -- L2/RConn1
  L2/LConn1 -- Current Sensor1/RConn2
  Diode/LConn1 -- Conn4/RConn1 -- Diode1/RConn1
  Diode/RConn1 -- Current Sensor2/LConn1 -- Conn2/RConn1 -- C8/LConn1
  Current Sensor1/LConn1 -- Conn1/RConn1
  Current Sensor1/RConn1 -- PS-Simulink Converter1/LConn1
  MOSFET 1/RConn1 -- Current Sensor2/RConn2
  MOSFET 2/RConn1 -- Current Sensor3/RConn2
  PS-Simulink Converter2/LConn1 -- Current Sensor2/RConn1
  PS-Simulink Converter3/LConn1 -- Current Sensor3/RConn1
  Simulink-PS Converter/RConn1 -- MOSFET 2/LConn1

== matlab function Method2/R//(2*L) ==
function y = fcn(Vout, Ton, Gv)

% current-sense resistor for the current transformer. 
%Here, Rsense here in the simulation is Ron of the MOSFET. Thus, Rsense = 0.01;
Rsense = 1;
L = 1e-3;

y = (Gv + Ton/(2*L)*Rsense)*Vout;

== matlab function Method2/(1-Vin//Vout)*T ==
function Ton = fcn(Vin, Vout)

T = 10e-6; 

Ton = ((Vout-Vin)/Vout)*T;
